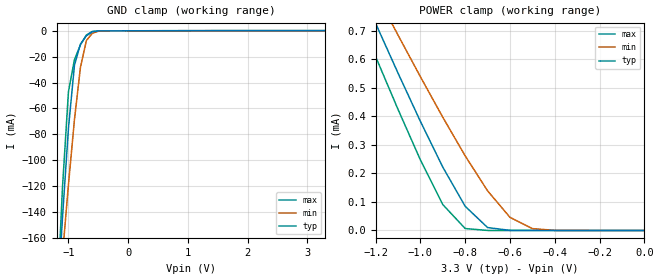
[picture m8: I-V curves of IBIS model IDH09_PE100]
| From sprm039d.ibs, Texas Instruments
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[Model]   IDH09_PE100
| Input with pulldown
Model_type   Input
Polarity   Non-Inverting
| signals   A, Y
Vinl = 0.8V
Vinh = 2.0V
|   typ   min   max
C_comp   1.5797p   1.5046p   1.7659p
|   typ   min   max
[Temperature Range]   25   -40   125
|   typ   min   max
[Voltage Range]   3.30V   3.00V   3.60V
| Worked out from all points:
|   GND clamp passes 1 mA (typ) near -0.61 V on its own axis
|   POWER clamp passes 1 mA (typ) near -1.35 V on its own axis
[GND_clamp]
|   Voltage   I(typ)   I(min)   I(max)
-3.3V     -2.003A    -1.514A    -2.598A
-1.2V     -221mA     -229.9mA   -219.1mA
-1.1V     -144.4mA   -173.2mA   -120.9mA
-1V       -75.23mA   -118.8mA   -46.95mA
-900mV    -26.63mA   -68.7mA    -22.36mA
-800mV    -10.29mA   -28.37mA   -10.92mA
-700mV    -3.831mA   -7.562mA   -3.281mA
-600mV    -789.8uA   -1.866mA   -448.7uA
-500mV    -112.8uA   -355.1uA   -87.29uA
-400mV    -39.84uA   -61.49uA   -56.21uA
3.3V      100.8uA    52.19uA    177.3uA
[POWER_clamp]
|   Voltage   I(typ)   I(min)   I(max)
-3.3V     4.588mA    4.102mA    4.731mA
-1.3V     903uA      983.5uA    798.1uA
-1.2V     725.8uA    833.2uA    609.3uA
-1.1V     551.6uA    684.6uA    424.5uA
-1V       382.2uA    538.7uA    247.4uA
-900mV    222.1uA    396.7uA    90.8uA
-800mV    84.67uA    261.3uA    6.783uA
-700mV    10.3uA     138.9uA    73.72nA
-600mV    329.7nA    46.05uA    888.2pA
-500mV    8.438nA    6.46uA     177.6pA
-400mV    355.3pA    466.6nA    177.6pA
0V        1pA        1pA        1pA
